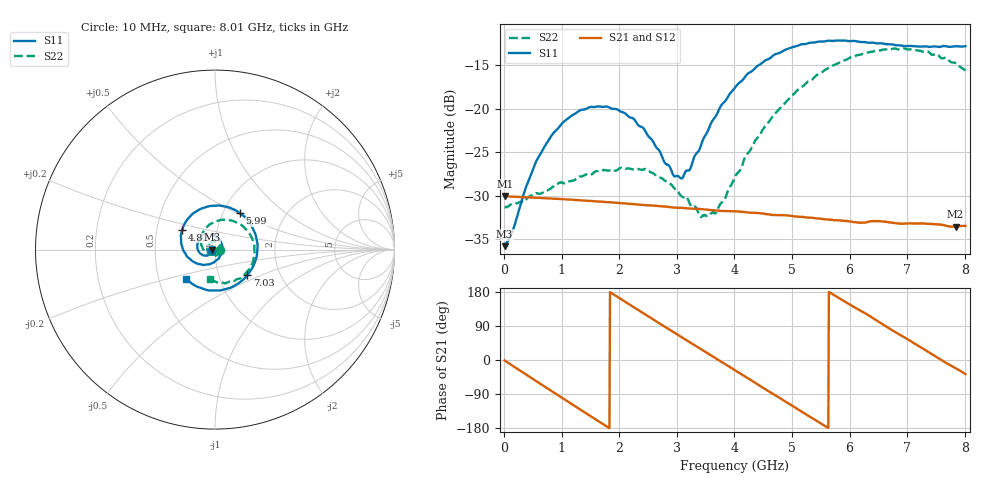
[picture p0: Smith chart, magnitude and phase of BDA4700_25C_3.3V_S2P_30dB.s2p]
!Agilent Technologies,E5071B,MY42404982,A.09.10
!Date: Mon Oct 20 18:15:41 2025
!Data & Calibration Information:
!Freq	S11:SOLT2(ON)	S21:SOLT2(ON)	S12:SOLT2(ON)	S22:SOLT2(ON)
# Hz S RI R 50
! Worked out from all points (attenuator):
!   801 points, 10 MHz to 8.01 GHz, reference 50 ohm
!   highest |S21| = -30.03 dB at 20 MHz (marker M1); lowest = -33.6 dB at 7.84 GHz (marker M2)
!   lowest |S11| = -35.8 dB at 10 MHz (marker M3), VSWR 1.03, Z = 48.4 - j0.104 ohm
!   |S11| at or under -10 dB: start of sweep to end of sweep
!   |S22| runs from -32.5 to -13.0 dB; largest |S21 - S12| = 0.0004
!   S11 on the Smith chart (normalised r, x): 10 MHz: 0.97, -0.00; 4.82 GHz: 0.68, +0.16; 5.99 GHz: 1.20, +0.52; 7.03 GHz: 1.37, -0.41; 8.01 GHz: 0.69, -0.24
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1e7  -0.0162 -0.00108  0.0315 -0.00066  0.0314 -0.000693  0.0271 -0.00082
2e7  -0.0165 -0.00178  0.0315 -0.00118  0.0314 -0.00131  0.0271 -0.00113
6e8  -0.041 -0.0334  0.0155 -0.0266  0.0155 -0.0265  0.0132 -0.0296
1.01e9  -0.0791 -0.0241  -0.00524 -0.0298  -0.00526 -0.0297  -0.0152 -0.0345
1.35e9  -0.0986 0.0078  -0.0204 -0.0216  -0.0204 -0.0217  -0.0365 -0.0183
2.08e9  -0.0497 0.0812  -0.0261 0.0116  -0.0261 0.0116  -0.0303 0.0337
2.68e9  0.0283 0.0508  -0.00404 0.0273  -0.0041 0.0272  0.0127 0.0384
2.95e9  0.0399 0.00987  0.00794 0.0259  0.00798 0.0258  0.0256 0.0239
3.09e9  0.0375 -0.0131  0.0136 0.0232  0.0134 0.0233  0.0285 0.0129
3.41e9  0.00742 -0.0598  0.0231 0.0131  0.0231 0.0131  0.0213 -0.0109
3.54e9  -0.0128 -0.0737  0.0251 0.00772  0.0251 0.00771  0.0143 -0.0195
3.69e9  -0.0419 -0.0824  0.0259 0.00141  0.026 0.00135  0.00169 -0.0254
4.01e9  -0.1107 -0.0726  0.0229 -0.0117  0.0229 -0.0116  -0.0309 -0.026
4.36e9  -0.1714 -0.0125  0.0125 -0.0218  0.0126 -0.0219  -0.0657 0.00108
4.82e9  -0.1815 0.1118  -0.00569 -0.0238  -0.00552 -0.0239  -0.0771 0.069
5.35e9  -0.0717 0.23  -0.0211 -0.0106  -0.021 -0.0107  -0.016 0.1465
5.99e9  0.1393 0.202  -0.019 0.0121  -0.0191 0.0121  0.1281 0.1478
6.68e9  0.2342 -0.0222  0.00234 0.022  0.00238 0.0221  0.2194 0.000653
7.03e9  0.1801 -0.1436  0.0133 0.0174  0.0134 0.0173  0.1992 -0.0931
7.46e9  0.0365 -0.226  0.0212 0.00466  0.0212 0.00471  0.111 -0.1727
7.84e9  -0.1089 -0.2019  0.0195 -0.0076  0.0195 -0.0077  0.0125 -0.1831
8.01e9  -0.1625 -0.1624  0.0169 -0.0128  0.0169 -0.0127  -0.0297 -0.1638
